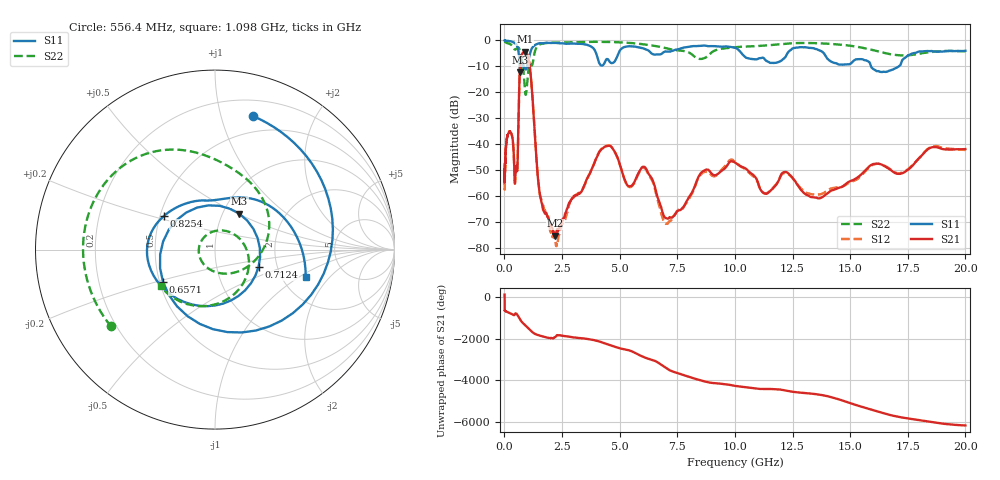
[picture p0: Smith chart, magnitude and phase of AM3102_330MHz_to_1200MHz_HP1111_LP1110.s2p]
! Date/Time: Tue, Sep 11, 2018 5:24 PM
! Network Analyzer: Agilent Technologies E8362B Rev: A.07.50.63
! Sweep from 0.010 to 20.000 GHz, 1601 Points, Sweep Type: LOG
! Power Supply: 4.949 V, 0.001 A
# Hz S DB R 50
!freq MagS11 AngS11 MagS21 AngS21 MagS12 AngS12 MagS22 AngS22
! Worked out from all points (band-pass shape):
!   1601 points, 10 MHz to 20 GHz, reference 50 ohm
!   highest |S21| = -4.26 dB at 886.4 MHz (marker M1); lowest = -75.3 dB at 2.207 GHz (marker M2)
!   |S21| within 3 dB of the highest: 706.9 MHz to 1.049 GHz (342.6 MHz wide, 39 % of centre)
!   lowest |S11| = -12.3 dB at 692.3 MHz (marker M3), VSWR 1.64, Z = 59.9 + j25.4 ohm
!   |S11| at or under -10 dB: 661.5 MHz to 738.9 MHz (77.41 MHz wide, 11.1 % of centre); 843.4 MHz to 983.1 MHz (139.7 MHz wide, 15.3 % of centre); 15.91 GHz to 17.11 GHz (1.201 GHz wide, 7.27 % of centre)
!   |S22| runs from -21.0 to -0.2 dB; largest |S21 - S12| = 0.0075
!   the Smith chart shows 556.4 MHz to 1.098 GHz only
!   S11 on the Smith chart (normalised r, x): 556.4 MHz: 0.34, +1.27; 657.1 MHz: 0.52, -0.21; 712.4 MHz: 1.60, -0.33; 825.4 MHz: 0.53, +0.22; 1.098 GHz: 2.68, -1.15
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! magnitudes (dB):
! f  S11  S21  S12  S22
! 10 MHz  0.0  -49.7  -47.4  -0.2
! 13.75 MHz  -0.1  -53.5  -57.0  -0.3
! 35.55 MHz  -0.1  -46.3  -46.2  -0.5
! 126.4 MHz  -0.2  -37.1  -37.0  -1.0
! 336.3 MHz  -0.6  -36.9  -36.7  -2.0
! 447.2 MHz  -1.0  -54.3  -54.1  -3.5
! 556.4 MHz  -2.2  -50.3  -50.2  -2.9
! 657.1 MHz  -9.4  -14.4  -14.5  -3.6
! 692.3 MHz  -12.3  -8.5  -8.5  -5.2
! 712.4 MHz  -11.7  -6.9  -7.0  -6.0
! 825.4 MHz  -9.4  -4.6  -4.6  -11.5
! 886.4 MHz  -10.9  -4.3  -4.4  -18.5
! 1.098 GHz  -5.5  -9.9  -9.8  -8.7
! 1.59 GHz  -1.1  -61.5  -61.0  -1.3
! 2.207 GHz  -0.9  -75.3  -77.4  -0.8
! 4.312 GHz  -9.2  -41.2  -40.9  -0.5
! 5.652 GHz  -2.4  -54.4  -54.6  -1.1
! 6.186 GHz  -3.6  -50.1  -50.5  -1.7
! 7.134 GHz  -4.3  -68.5  -69.8  -3.3
! 9.761 GHz  -2.4  -47.0  -46.2  -2.8
! 13.55 GHz  -3.3  -60.6  -59.4  -1.1
! 20 GHz  -4.0  -41.9  -42.2  -4.2
